|   IBIS file stm32l471_476_486_ufbga132.ibs
[IBIS ver]   4.2
[File name]   stm32l471_476_486_ufbga132.ibs
[File Rev]   3.0
[Date]   08-10-2018
[Source]   Data Created at STMicroelectronics
[Notes]   File originated from ELDO simulations.
[Disclaimer]  This information is for modeling purpose only and is
   not guaranteed.
   The information is subject to change without notice.
[Copyright]   Copyright 2018 STMicroelectronics Inc.
|   Component stm32l471_476_486_ufbga132
[Component] stm32l471_476_486_ufbga132
[Manufacturer] STMicroelectronics
[Package]
| variable   typ   min   max
R_pkg   0.0   0.0   0.0
L_pkg   0.0H   0.0H   0.0H
C_pkg   0.0F   0.0F   0.0F
[Pin]  signal_name   model_name   R_pin   L_pin   C_pin
A1 PE3 io8prog2m25m50m120m_sudq_ft
A10 PA14 io8prog2m25m50m120m_sudq_ft
A11 PA13 io8prog2m25m50m120m_sudq_ft
A12 PA12 io8usblsfs_otg2
A2 PE1 io8prog2m25m50m120m_sudq_ft
A3 PB8 io8prog2m25m50m120m_sudq_i2c_ft
A4 BOOT0 vpp_test_hv
A5 PD7 io8prog2m25m50m120m_sudq_ft
A6 PD5 io8prog2m25m50m120m_sudq_ft
A7 PB4 io8prog2m25m50m120m_sudq_ft
A8 PB3 io8prog2m25m50m120m_sudq_ft
A9 PA15 io8prog2m25m50m120m_sudq_ft
B1 PE4 io8prog2m25m50m120m_sudq_ft
B10 PC12 io8prog2m25m50m120m_sudq_ft
B11 PC10 io8prog2m25m50m120m_sudq_ft
B12 PA11 io8usblsfs_otg2
B2 PE2 io8prog2m25m50m120m_sudq_ft
B3 PB9 io8prog2m25m50m120m_sudq_i2c_ft
B4 PB7 io8prog2m25m50m120m_sudq_i2c_ft
B5 PB6 io8prog2m25m50m120m_sudq_i2c_ft
B6 PD6 io8prog2m25m50m120m_sudq_ft
B7 PD4 io8prog2m25m50m120m_sudq_ft
B8 PD3 io8prog2m25m50m120m_sudq_ft
B9 PD1 io8prog2m25m50m120m_sudq_ft
C1 PC13 io8prog2m25m50m120m_sudq_ft
C10 PC11 io8prog2m25m50m120m_sudq_ft
C11 VDDUSB/VDD POWER
C12 PA10 io8usb_id_otg20_lcd4_ft_ms
C2 PE5 io8prog2m25m50m120m_sudq_ft
C3 PE0 io8prog2m25m50m120m_sudq_ft
C4 VDD POWER
C5 PB5 io8prog2m25m50m120m_sudq_ft
C6 PG14 io8prog2m25m50m120m_sudq_i2c_ft
C7 PG13 io8prog2m25m50m120m_sudq_i2c_ft
C8 PD2 io8prog2m25m50m120m_sudq_ft
C9 PD0 io8prog2m25m50m120m_sudq_ft
D1 PC14-OSC32_IN io8prog2m25m50m120m_sudq_ft
D10 PA9 POWER
D11 PA8 io8prog2m25m50m120m_sudq_ft
D12 PC9 io8prog2m25m50m120m_sudq_ft
D2 PE6 io8prog2m25m50m120m_sudq_ft
D3 VSS GND
D4 PF2 io8prog2m25m50m120m_sudq_ft
D5 PF1 io8prog2m25m50m120m_sudq_i2c_ft
D6 PF0 io8prog2m25m50m120m_sudq_i2c_ft
D7 PG12 io8prog2m25m50m120m_sudq_ft
D8 PG10 io8prog2m25m50m120m_sudq_ft
D9 PG9 io8prog2m25m50m120m_sudq_ft
E1 PC15-OSC32_OUT io8prog2m25m50m120m_sudq_ft
E10 PC8 io8prog2m25m50m120m_sudq_ft
E11 PC7 io8prog2m25m50m120m_sudq_ft
E12 PC6 io8prog2m25m50m120m_sudq_ft
E2 VBAT POWER
E3 VSS GND
E4 PF3 io8prog2m25m50m120m_sudq_ft
E9 PG5 io8prog2m25m50m120m_sudq_ft
F1 PH0-OSC_IN io8prog2m25m50m120m_sudq_ft
F10 PG4 io8prog2m25m50m120m_sudq_ft
F11 VSS GND
F12 VSS GND
F2 VSS GND
F3 PF4 io8prog2m25m50m120m_sudq_ft
F4 PF5 io8prog2m25m50m120m_sudq_ft
F6 VSS GND
F7 VSS GND
F9 PG3 io8prog2m25m50m120m_sudq_ft
G1 PH1-OSC_OUT io8prog2m25m50m120m_sudq_ft
G10 PG2 io8prog2m25m50m120m_sudq_ft
G11 VDD POWER
G12 VDD POWER
G2 VDD POWER
G3 PG11 io8prog2m25m50m120m_sudq_ft
G4 PG6 io8prog2m25m50m120m_sudq_ft
G6 VDD POWER
G7 VDDIO2 POWER
G9 PG1 io8prog2m25m50m120m_sudq_ft
H1 PC0 io8prog2m25m50m120m_sudq_i2c_ft
H10 PD15 io8prog2m25m50m120m_sudq_ft
H11 PD14 io8prog2m25m50m120m_sudq_ft
H12 PD13 io8prog2m25m50m120m_sudq_ft
H2 NRST ioreset_ft_v33
H3 VDD POWER
H4 PG7 io8prog2m25m50m120m_sudq_i2c_ft
H9 PG0 io8prog2m25m50m120m_sudq_ft
J1 VSSA_VREF- GND
J10 PD12 io8prog2m25m50m120m_sudq_ft
J11 PD11 io8prog2m25m50m120m_sudq_ft
J12 PD10 io8prog2m25m50m120m_sudq_ft
J2 PC1 io8prog2m25m50m120m_sudq_i2c_ft
J3 PC2 io8prog2m25m50m120m_sudq_ft
J4 PA4 io8prog2m25m50m120m_sudq_ft
J5 PA7 io8prog2m25m50m120m_sudq_ft
J6 PG8 io8prog2m25m50m120m_sudq_i2c_ft
J7 PF12 io8prog2m25m50m120m_sudq_ft
J8 PF14 io8prog2m25m50m120m_sudq_ft
J9 PF15 io8prog2m25m50m120m_sudq_ft
K1 PG15 io8prog2m25m50m120m_sudq_ft
K10 PB15 io8prog2m25m50m120m_sudq_ft
K11 PB14 io8prog2m25m50m120m_sudq_i2c_ft
K12 PB13 io8prog2m25m50m120m_sudq_i2c_ft
K2 PC3 io8prog2m25m50m120m_sudq_ft
K3 PA2 io8prog2m25m50m120m_sudq_ft
K4 PA5 io8prog2m25m50m120m_sudq_ft
K5 PC4 io8prog2m25m50m120m_sudq_ft
K6 PF11 io8prog2m25m50m120m_sudq_ft
K7 PF13 io8prog2m25m50m120m_sudq_ft
K8 PD9 io8prog2m25m50m120m_sudq_ft
K9 PD8 io8prog2m25m50m120m_sudq_ft
L1 VREF+ POWER
L10 PB10 io8prog2m25m50m120m_sudq_i2c_ft
L11 PB11 io8prog2m25m50m120m_sudq_i2c_ft
L12 PB12 io8w_swp_lcd4_ft
L2 PA0 io8prog2m25m50m120m_sudq_ft
L3 PA3 io8prog2m25m50m120m_sudq_ft
L4 PA6 io8prog2m25m50m120m_sudq_ft
L5 PC5 io8prog2m25m50m120m_sudq_ft
L6 PB2 io8prog2m25m50m120m_sudq_ft
L7 PE8 io8prog2m25m50m120m_sudq_ft
L8 PE10 io8prog2m25m50m120m_sudq_ft
L9 PE12 io8prog2m25m50m120m_sudq_ft
M1 VDDA POWER
M10 PE13 io8prog2m25m50m120m_sudq_ft
M11 PE14 io8prog2m25m50m120m_sudq_ft
M12 PE15 io8prog2m25m50m120m_sudq_ft
M2 PA1 io8prog2m25m50m120m_sudq_ft
M3 OPAMP1_VINM NC
M4 OPAMP2_VINM NC
M5 PB0 io8prog2m25m50m120m_sudq_ft
M6 PB1 io8prog2m25m50m120m_sudq_ft
M7 PE7 io8prog2m25m50m120m_sudq_ft
M8 PE9 io8prog2m25m50m120m_sudq_ft
M9 PE11 io8prog2m25m50m120m_sudq_ft
[Model Selector] io8prog2m25m50m120m_sudq_ft
iols8p_sudq_ft_pd_lv  "IO low speed, PD=40kOhm - 1P8V"
iols8p_sudq_ft_pu_lv  "IO low speed, PU=40kOhm - 1P8V"
iols8p_sudq_ft_lv  "IO low speed - 1P8V"
iols8p_sudq_ft_pd  "IO low speed, PD=40kOhm - 3P3V"
iols8p_sudq_ft_pu  "IO low speed, PU=40kOhm - 3P3V"
iols8p_sudq_ft  "IO low speed - 3P3V"
iofs8p_sudq_ft_pd_lv  "IO full speed, PD=40kOhm - 1P8V"
iofs8p_sudq_ft_pu_lv  "IO full speed, PU=40kOhm - 1P8V"
iofs8p_sudq_ft_lv  "IO full speed - 1P8V"
iofs8p_sudq_ft_pd  "IO full speed, PD=40kOhm - 3P3V"
iofs8p_sudq_ft_pu  "IO full speed, PU=40kOhm - 3P3V"
iofs8p_sudq_ft  "IO full speed - 3P3V"
ioms8p_sudq_ft_pd_lv  "IO medium speed, PD=40kOhm - 1P8V"
ioms8p_sudq_ft_pu_lv  "IO medium speed, PU=40kOhm - 1P8V"
ioms8p_sudq_ft_lv  "IO medium speed - 1P8V"
ioms8p_sudq_ft_pd  "IO medium speed, PD=40kOhm - 3P3V"
ioms8p_sudq_ft_pu  "IO medium speed, PU=40kOhm - 3P3V"
ioms8p_sudq_ft  "IO medium speed - 3P3V"
iohs8p_sudq_ft_pd_lv  "IO high speed, PD=40kOhm - 1P8V"
iohs8p_sudq_ft_pu_lv  "IO high speed, PU=40kOhm - 1P8V"
iohs8p_sudq_ft_lv  "IO high speed - 1P8V"
iohs8p_sudq_ft_pd  "IO high speed, PD=40kOhm - 3P3V"
iohs8p_sudq_ft_pu  "IO high speed, PU=40kOhm - 3P3V"
iohs8p_sudq_ft  "IO high speed - 3P3V"
[Model Selector] io8prog2m25m50m120m_sudq_i2c_ft
io8prog_1v8_i2c_pd  "5V Tol GPIO 1.8V range i2c functionality with pull down"
io8prog_1v8_i2c_pu  "5V Tol GPIO 1.8V range i2c functionality with pull up"
io8prog_1v8_i2c  "5V Tol GPIO 1.8V range i2c functionality"
io8prog_3v3_i2c_pd  "5V Tol GPIO 3.3V range i2c functionality with pull down"
io8prog_3v3_i2c_pu  "5V Tol GPIO 3.3V range i2c functionality with pull up"
io8prog_3v3_i2c  "5V Tol GPIO 3.3V range i2c functionality"
io8ls_1v8_pd  "5V Tol GPIO 1.8V range with pd io low speed"
io8ls_1v8_pu  "5V Tol GPIO 1.8V range with pu io low speed"
io8ls_1v8  "5V Tol GPIO 1.8V range io low speed"
io8ls_3v3_pd  "5V Tol GPIO 3.3V range with pd io low speed"
io8ls_3v3_pu  "5V Tol GPIO 3.3V range with pu io low speed"
io8ls_3v3  "5V Tol GPIO 3.3V range io low speed"
io8fs_1v8_pd  "5V Tol GPIO 1.8V range with pd io full speed"
io8fs_1v8_pu  "5V Tol GPIO 1.8V range with pu io full speed"
io8fs_1v8  "5V Tol GPIO 1.8V range io full speed"
io8fs_3v3_pd  "5V Tol GPIO 3.3V range with pd io full speed"
io8fs_3v3_pu  "5V Tol GPIO 3.3V range with pu io full speed"
io8fs_3v3  "5V Tol GPIO 3.3V range io full speed"
io8ms_1v8_pd  "5V Tol GPIO 1.8V range with pd io medium speed"
io8ms_1v8_pu  "5V Tol GPIO 1.8V range with pu io medium speed"
io8ms_1v8  "5V Tol GPIO 1.8V range io medium speed"
io8ms_3v3_pd  "5V Tol GPIO 3.3V range with pd io medium speed"
io8ms_3v3_pu  "5V Tol GPIO 3.3V range with pu io medium speed"
io8ms_3v3  "5V Tol GPIO 3.3V range io medium speed"
io8hs_1v8_pd  "5V Tol GPIO 1.8V range with pd io high speed"
io8hs_1v8_pu  "5V Tol GPIO 1.8V range with pu io high speed"
io8hs_1v8  "5V Tol GPIO 1.8V range io high speed"
io8hs_3v3_pd  "5V Tol GPIO 3.3V range with pd io high speed"
io8hs_3v3_pu  "5V Tol GPIO 3.3V range with pu io high speed"
io8hs_3v3  "5V Tol GPIO 3.3V range io high speed"
[Model Selector] io8usb_id_otg20_lcd4_ft_ms
io8usbid_1v8_id_pu  "ID 1V8 range with pull up"
io8usbid_3v3_id_pu  "ID 3V3 range with pull up"
io8usbid_1v8_id  "ID 1V8 range"
io8usbid_3v3_id  "ID 3V3 range"
io8lsusbid_1v8_pd  "GPIO 1.8V range with pd io low speed"
io8lsusbid_1v8_pu  "GPIO 1.8V range with pu io low speed"
io8lsusbid_1v8  "GPIO 1.8V range io low speed"
io8lsusbid_3v3_pd  "GPIO 3.3V range with pd io low speed"
io8lsusbid_3v3_pu  "GPIO 3.3V range with pu io low speed"
io8lsusbid_3v3  "GPIO 3.3V range io low speed"
io8fsusbid_1v8_pd  "GPIO 1.8V range with pd io full speed"
io8fsusbid_1v8_pu  "GPIO 1.8V range with pu io full speed"
io8fsusbid_1v8  "GPIO 1.8V range io full speed"
io8fsusbid_3v3_pd  "GPIO 3.3V range with pd io full speed"
io8fsusbid_3v3_pu  "GPIO 3.3V range with pu io full speed"
io8fsusbid_3v3  "GPIO 3.3V range io full speed"
io8msusbid_1v8_pd  "GPIO 1.8V range with pd io medium speed"
io8msusbid_1v8_pu  "GPIO 1.8V range with pu io medium speed"
io8msusbid_1v8  "GPIO 1.8V range io medium speed"
io8msusbid_3v3_pd  "GPIO 3.3V range with pd io medium speed"
io8msusbid_3v3_pu  "GPIO 3.3V range with pu io medium speed"
io8msusbid_3v3  "GPIO 3.3V range io medium speed"
io8hsusbid_1v8_pd  "GPIO 1.8V range with pd io high speed"
io8hsusbid_1v8_pu  "GPIO 1.8V range with pu io high speed"
io8hsusbid_1v8  "GPIO 1.8V range io high speed"
io8hsusbid_3v3_pd  "GPIO 3.3V range with pd io high speed"
io8hsusbid_3v3_pu  "GPIO 3.3V range with pu io high speed"
io8hsusbid_3v3  "GPIO 3.3V range io high speed"
[Model Selector] io8usblsfs_otg2
usb_ls_pd  "USB Low Speed mode - Pull Down"
usb_ls_pu2  "USB Low Speed mode - Pull up 2"
usb_ls_pu  "USB Low Speed mode - Pull up"
usb_fs  "USB Low Speed mode"
usb_fs_pd  "USB Full Speed mode - Pull Down"
usb_fs_pu2  "USB Full Speed mode - Pull up 2"
usb_fs_pu  "USB Full Speed mode - Pull up"
[Model Selector] ioreset_ft_v33
ioreset_1v2_pu  "RESET 1.2V range with PU"
ioreset_1v2  "RESET 1.2V range"
ioreset_1v8_pu  "RESET 1.8V range with PU"
ioreset_1v8  "RESET 1.8V range"
ioreset_3v3_pu  "RESET 3.3V range with PU"
ioreset_3v3  "RESET 3.3V range"
[Model Selector] io8w_swp_lcd4_ft
io8w_swp_classc  "Class C swp functionality"
io8w_swp_classb  "Class B swp functionality"
io8lsw_1v8_pd  "GPIO 1.8V range with pd io low speed"
io8lsw_1v8_pu  "GPIO 1.8V range with pu io low speed"
io8lsw_1v8  "GPIO 1.8V range io low speed"
io8lsw_3v3_pd  "GPIO 3.3V range with pd io low speed"
io8lsw_3v3_pu  "GPIO 3.3V range with pu io low speed"
io8lsw_3v3  "GPIO 3.3V range io low speed"
io8fsw_1v8_pd  "GPIO 1.8V range with pd io full speed"
io8fsw_1v8_pu  "GPIO 1.8V range with pu io full speed"
io8fsw_1v8  "GPIO 1.8V range io full speed"
io8fsw_3v3_pd  "GPIO 3.3V range with pd io full speed"
io8fsw_3v3_pu  "GPIO 3.3V range with pu io full speed"
io8fsw_3v3  "GPIO 3.3V range io full speed"
io8msw_1v8_pd  "GPIO 1.8V range with pd io medium speed"
io8msw_1v8_pu  "GPIO 1.8V range with pu io medium speed"
io8msw_1v8  "GPIO 1.8V range io medium speed"
io8msw_3v3_pd  "GPIO 3.3V range with pd io medium speed"
io8msw_3v3_pu  "GPIO 3.3V range with pu io medium speed"
io8msw_3v3  "GPIO 3.3V range io medium speed"
io8hsw_1v8_pd  "GPIO 1.8V range with pd io high speed"
io8hsw_1v8_pu  "GPIO 1.8V range with pu io high speed"
io8hsw_1v8  "GPIO 1.8V range io high speed"
io8hsw_3v3_pd  "GPIO 3.3V range with pd io high speed"
io8hsw_3v3_pu  "GPIO 3.3V range with pu io high speed"
io8hsw_3v3  "GPIO 3.3V range io high speed"
[Model Selector] vpp_test_hv
vpp_1v8  "VPP with test functionality 1.8V range"
vpp_3v3  "VPP with test functionality 3.3V range"
| Models and submodels in the file (123): iols8p_sudq_ft_pd_lv (I/O), iols8p_sudq_ft_pu_lv (I/O), iols8p_sudq_ft_lv (I/O), iols8p_sudq_ft_pd (I/O), iols8p_sudq_ft_pu (I/O), iols8p_sudq_ft (I/O), iofs8p_sudq_ft_pd_lv (I/O), iofs8p_sudq_ft_pu_lv (I/O), iofs8p_sudq_ft_lv (I/O), iofs8p_sudq_ft_pd (I/O), iofs8p_sudq_ft_pu (I/O), iofs8p_sudq_ft (I/O), ioms8p_sudq_ft_pd_lv (I/O), ioms8p_sudq_ft_pu_lv (I/O), ioms8p_sudq_ft_lv (I/O), ioms8p_sudq_ft_pd (I/O), ioms8p_sudq_ft_pu (I/O), ioms8p_sudq_ft (I/O), iohs8p_sudq_ft_pd_lv (I/O), iohs8p_sudq_ft_pu_lv (I/O), iohs8p_sudq_ft_lv (I/O), iohs8p_sudq_ft_pd (I/O), iohs8p_sudq_ft_pu (I/O), iohs8p_sudq_ft (I/O), io8prog_1v8_i2c_pd (I/O), io8prog_1v8_i2c_pu (I/O), io8prog_1v8_i2c (I/O), io8prog_3v3_i2c_pd (I/O), io8prog_3v3_i2c_pu (I/O), io8prog_3v3_i2c (I/O), io8ls_1v8_pd (I/O), io8ls_1v8_pu (I/O), io8ls_1v8 (I/O), io8ls_3v3_pd (I/O), io8ls_3v3_pu (I/O), io8ls_3v3 (I/O), io8fs_1v8_pd (I/O), io8fs_1v8_pu (I/O), io8fs_1v8 (I/O), io8fs_3v3_pd (I/O), io8fs_3v3_pu (I/O), io8fs_3v3 (I/O), io8ms_1v8_pd (I/O), io8ms_1v8_pu (I/O), io8ms_1v8 (I/O), io8ms_3v3_pd (I/O), io8ms_3v3_pu (I/O), io8ms_3v3 (I/O), io8hs_1v8_pd (I/O), io8hs_1v8_pu (I/O), io8hs_1v8 (I/O), io8hs_3v3_pd (I/O), io8hs_3v3_pu (I/O), io8hs_3v3 (I/O), io8usbid_1v8_id_pu (Input), io8usbid_3v3_id_pu (Input), io8usbid_1v8_id (Input), io8usbid_3v3_id (Input), io8lsusbid_1v8_pd (I/O), io8lsusbid_1v8_pu (I/O), io8lsusbid_1v8 (I/O), io8lsusbid_3v3_pd (I/O), io8lsusbid_3v3_pu (I/O), io8lsusbid_3v3 (I/O), io8fsusbid_1v8_pd (I/O), io8fsusbid_1v8_pu (I/O), io8fsusbid_1v8 (I/O), io8fsusbid_3v3_pd (I/O), io8fsusbid_3v3_pu (I/O), io8fsusbid_3v3 (I/O), io8msusbid_1v8_pd (I/O), io8msusbid_1v8_pu (I/O), io8msusbid_1v8 (I/O), io8msusbid_3v3_pd (I/O), io8msusbid_3v3_pu (I/O), io8msusbid_3v3 (I/O), io8hsusbid_1v8_pd (I/O), io8hsusbid_1v8_pu (I/O), io8hsusbid_1v8 (I/O), io8hsusbid_3v3_pd (I/O)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
